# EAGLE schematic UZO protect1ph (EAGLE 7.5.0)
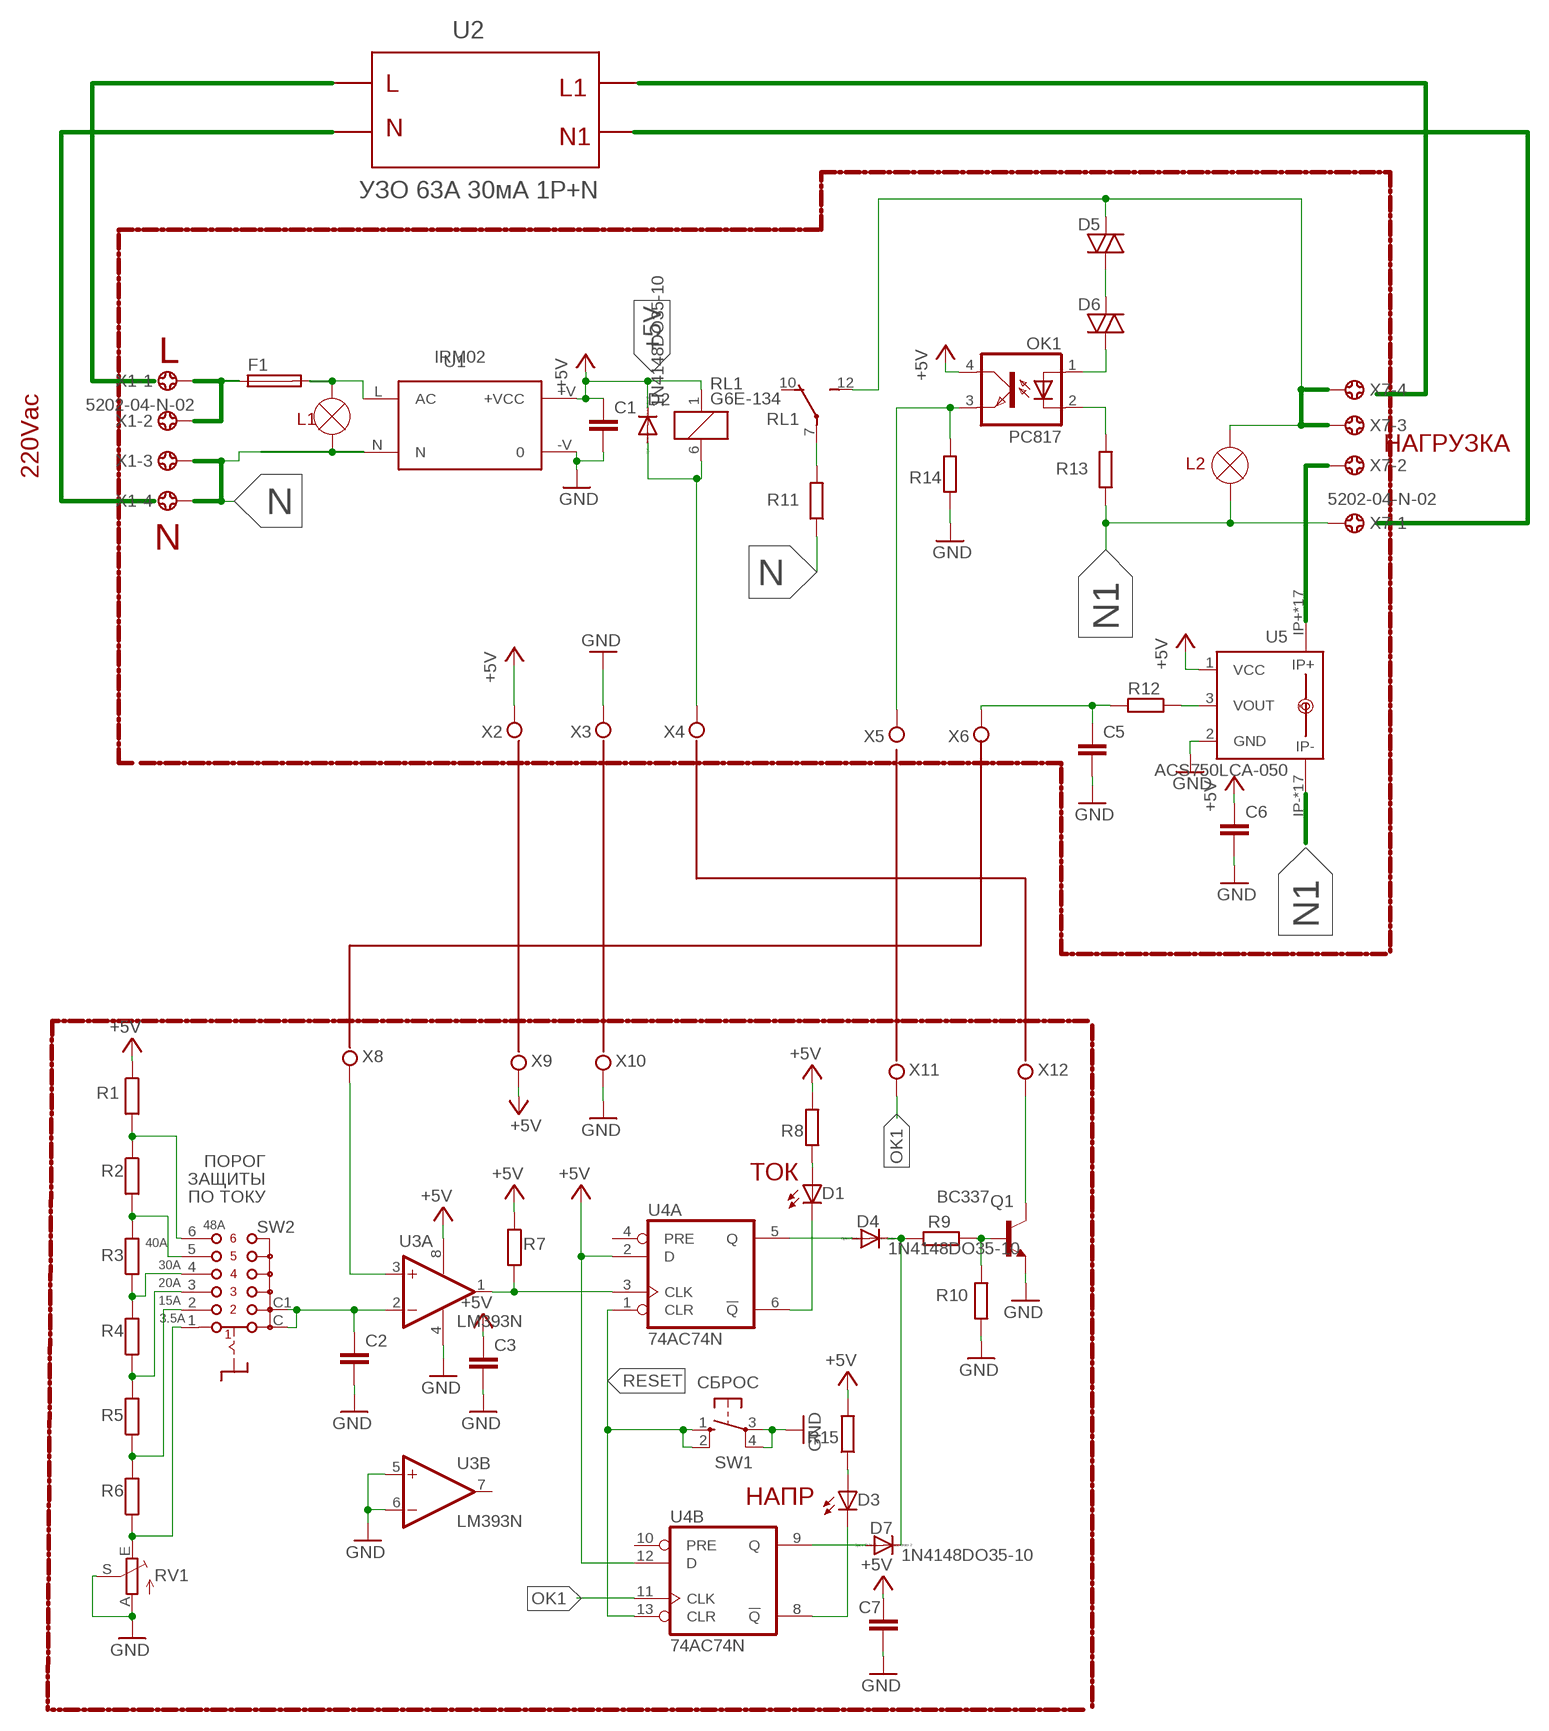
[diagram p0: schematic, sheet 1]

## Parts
C1  C-EUC1206  [C1206]
C2  C-EUC1206  [C1206]
C3  C-EUC1206  [C1206]
C5  C-EUC1206  [C1206]
C6  C-EUC1206  [C1206]
D1  LED5MM  [LED5MM]
D2  1N4148DO35-10  [DO35-10]
D3  LED5MM  [LED5MM]
D4  1N4148DO35-10  [DO35-10]
D5  DIAC-DO35-10  [DO35-10]
D6  DIAC-DO35-10  [DO35-10]
D7  1N4148DO35-10  [DO35-10]
F1  FUSEGSH15 1A 5x20mm  FUSEGSH15  [GSH15]
OK1  PC817  [DIL04]
Q1  BC337  [TO92]
R1  R-EU_R1206  [R1206]
R2  R-EU_R1206  [R1206]
R3  R-EU_R1206  [R1206]
R4  R-EU_R1206  [R1206]
R5  R-EU_R1206  [R1206]
R6  R-EU_R1206  [R1206]
R7  R-EU_R1206  [R1206]
R8  R-EU_R1206  [R1206]
R9  R-EU_R1206  [R1206]
R10  R-EU_R1206  [R1206]
R11  R-EU_0817/22  [P0817/22]
R12  R-EU_R1206  [R1206]
R13  R-EU_0817/22  [P0817/22]
R14  R-EU_R1206  [R1206]
R15  R-EU_R1206  [R1206]
RL1  G6E-134  [G6E]
RV1  TRIM_EU-RS3  [RS3]
SW1  SPST Push Button  10-XX  [B3F-10XX]
SW2  SS-10-16  [SS-10-16]
U1  IRM02  [IRM02]
U3  LM393N  [DIL08]
U4  74AC74N  [DIL14]
U5  ACS750LCA-050  [ACS75050]
X1  5202-04-N-02  [5202-04-N-02]
X2  TPPAD1-17  [P1-17]
X3  TPPAD1-17  [P1-17]
X4  TPPAD1-17  [P1-17]
X5  TPPAD1-17  [P1-17]
X6  TPPAD1-17  [P1-17]
X7  5202-04-N-02  [5202-04-N-02]
X8  TPPAD1-17  [P1-17]
X9  TPPAD1-17  [P1-17]
X10  TPPAD1-17  [P1-17]
X11  TPPAD1-17  [P1-17]
X12  TPPAD1-17  [P1-17]
С7  C-EUC1206  [C1206]

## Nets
+5V: C1.1 C3.1 C6.1 D2.C OK1.4(COL) R1.1 R7.1 R8.2 R15.2 RL1.1 U1.+V(+VCC) U3.8(P:V+) U4.2(A:D) U4.12(B:D) U5.1(VCC) X2.TP X9.TP С7.1
GND: C1.2 C2.2 C3.2 C5.2 C6.2 Q1.1(E) R10.2 R14.1 RV1.A RV1.S SW1.3(P) SW1.4(P1) U1.-V U3.4(P:V-) U3.5(B:+IN) U3.6(B:-IN) U5.2(GND) X3.TP X10.TP С7.2
N: R11.1 U1.N X1.3 X1.4
N1: R13.1 U5.IP- U5.IP-@2(IP-) U5.IP-@3(IP-) U5.IP-@4(IP-) U5.IP-@5(IP-) U5.IP-@6(IP-) U5.IP-@7(IP-) U5.IP-@8(IP-) U5.IP-@9(IP-) U5.IP-@10(IP-) U5.IP-@11(IP-) U5.IP-@12(IP-) U5.IP-@13(IP-) U5.IP-@14(IP-) U5.IP-@15(IP-) U5.IP-@16(IP-) U5.IP-@17(IP-) X7.1
N$1: F1.1 X1.1 X1.2
N$2: R11.2 RL1.7(P)
N$3: F1.2 U1.L(AC)
N$4: D2.A RL1.6 X4.TP
N$5: U5.IP+ U5.IP+@2(IP+) U5.IP+@3(IP+) U5.IP+@4(IP+) U5.IP+@5(IP+) U5.IP+@6(IP+) U5.IP+@7(IP+) U5.IP+@8(IP+) U5.IP+@9(IP+) U5.IP+@10(IP+) U5.IP+@11(IP+) U5.IP+@12(IP+) U5.IP+@13(IP+) U5.IP+@14(IP+) U5.IP+@15(IP+) U5.IP+@16(IP+) U5.IP+@17(IP+) X7.2
N$6: U3.3(A:+IN) X8.TP
N$7: X7.4
N$8: D5.A D6.C
N$9: D6.A OK1.1(A)
N$10: OK1.2(C) R13.2
N$11: OK1.3(EMIT) R14.2 X5.TP
N$12: R12.1 U5.3(VOUT)
N$13: C5.1 R12.2 X6.TP
N$16: D5.C RL1.12(S) X7.3
N$17: R7.2 U3.1(A:OUT) U4.3(A:CLK)
N$20: R1.2 R2.1 SW2.6
N$21: R3.1 R4.2 SW2.4
N$22: R2.2 R3.2 SW2.5
N$23: C2.1 SW2.C SW2.C1 U3.2(A:-IN)
N$24: R4.1 R5.2 SW2.3
N$25: D1.A R8.1
N$26: R5.1 R6.2 SW2.2
N$27: D3.A R15.1
N$28: Q1.2(B) R9.1 R10.1
N$29: R6.1 RV1.E SW2.1
N$30: D4.A U4.5(A:Q)
N$31: D4.C D7.C R9.2
N$32: D7.A U4.9(B:Q)
N$33: Q1.3(C) X12.TP
OK1: U4.11(B:CLK) X11.TP
PB1: D3.K(C) U4.8(B:!Q)
PB4: D1.K(C) U4.6(A:!Q)
RESET: SW1.1(S) SW1.2(S1) U4.1(A:CLR) U4.13(B:CLR)
Unconnected: RL1.10(O) U3.7(B:OUT) U4.4(A:PRE) U4.10(B:PRE)

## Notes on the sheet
- U2
- L | L1
- N
- N1
- УЗО 63А 30мА 1Р+N
- L
- L1
- НАГРУЗКА
- L2
- 220Vac
- N
- ПОРОГ
- ЗАЩИТЫ | ТОК
- ПО ТОКУ
- 48A
- 40A
- 30A
- 20A
- 15A
- 3.5A
- СБРОС
- НАПР

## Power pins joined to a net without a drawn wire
GND: U4.7(P:GND)
VCC: U4.14(P:VCC)

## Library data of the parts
C1-C3 C5 C6 С7 = rcl:C-EU: CAPACITOR, European symbol
D1 D3 = led:LED: LED
D2 D4 D7 = diode:1N4148: DIODE
D5 D6 = diode:DIAC-: DIAC
F1 = fuse:FUSE: Fuse; OC_FARNELL: unknown; OC_NEWARK: unknown
OK1 = optocoupler:PC817: SHARP OPTO COUPLER; MPN: PC817X4J000F; OC_FARNELL: 9707727; OC_NEWARK: 97K7059
Q1 = transistor:BC337: NPN TRANSISTOR
R1-R15 = rcl:R-EU_: RESISTOR, European symbol
RL1 = relay:G6E-134
RV1 = pot:TRIM_EU-: POTENTIOMETER
SW1 = switch-omron:10-XX: OMRON SWITCH; MPN: B3F-1000; OC_FARNELL: 176432; OC_NEWARK: 36M3542
SW2 = switch:SS-10-16: Rotary Switch, Through Hole, 6 Position, 1 Pole
U1 = acdc:IRM02: 2W Single Output ACDC converter
U3 = linear:LM393: COMPARATOR
U4 = 74xx-eu:74*74: Dual D type positive edge triggered FLIP FLOP, preset and clear
U5 = allegro:ACS750*CA-050: Current Sensor display layer 49 Reference in BRD and place VIAs on circles Source: www.allegromicro.com/datafile/0750-050.pdf; MF: ALLEGRO MICROSYSTEMS, INC.; MPN: ACS750LCA-050; OC_FARNELL: 1457176; OC_NEWARK: 61H4464
X1 X7 = con-ebyelectro:5202-04-N-02: Barrier Blocks Sreies 5202 Source: http://www.ebyelectro.com/PDF/5202-XX-N-02.pdf; OC_FARNELL: unknown; OC_NEWARK: unknown
X2-X6 X8-X12 = testpad:TP: Test pad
